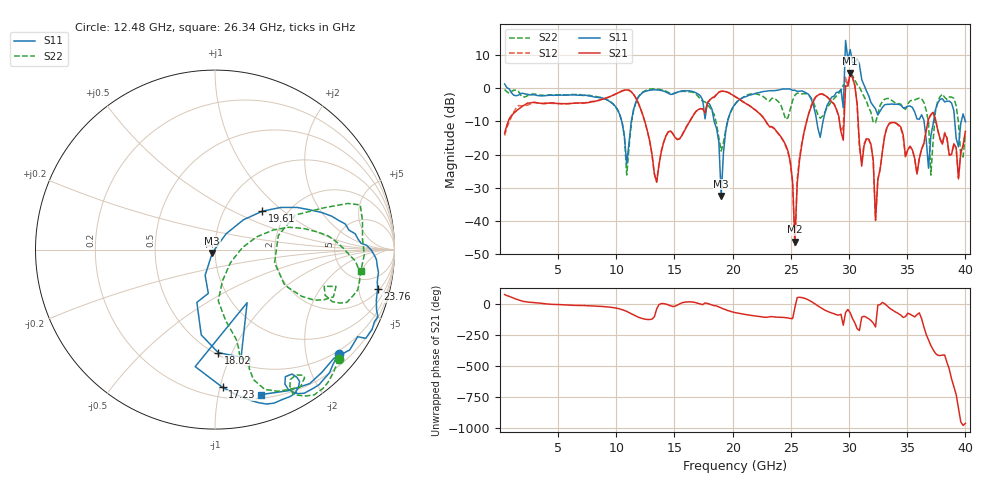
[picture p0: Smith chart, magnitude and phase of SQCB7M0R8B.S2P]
! Network Analyzer HP8722ES.07.66: Jul 25, 2000 Serial No. US39175408
! 26 Oct 2004  10:26:45
! Frequency  S11  S21  S12  S22
# HZ  S  DB R  50
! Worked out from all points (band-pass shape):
!   201 points, 400 MHz to 40 GHz, reference 50 ohm
!   highest |S21| = 4.62 dB at 30.1 GHz (marker M1); lowest = -46.3 dB at 25.35 GHz (marker M2)
!   |S21| within 3 dB of the highest: 29.95 GHz to 30.44 GHz (487.3 MHz wide, 1.61 % of centre)
!   lowest |S11| = -32.5 dB at 19.01 GHz (marker M3), VSWR 1.05, Z = 48.5 - j1.77 ohm
!   |S11| at or under -10 dB: 10.47 GHz to 11.29 GHz (819.6 MHz wide, 7.53 % of centre); 18.41 GHz to 19.57 GHz (1.159 GHz wide, 6.1 % of centre); 36.45 GHz to 37.26 GHz (812.6 MHz wide, 2.2 % of centre)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
!   |S22| runs from -26.2 to 3.9 dB; largest |S21 - S12| = 0.62
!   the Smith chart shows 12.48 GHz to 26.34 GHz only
!   S11 on the Smith chart (normalised r, x): 12.48 GHz: 0.43, -2.67; 17.23 GHz: 0.27, -1.02; 18.02 GHz: 0.52, -0.89; 19.61 GHz: 1.51, +0.73; 23.76 GHz: 2.25, -7.65; 26.34 GHz: 0.23, -1.34
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4e8  1.30 -15.1  -13.48 75.8  -14.23 80.6  -0.38 -7.8
7.132e9  -2.14 -101.7  -4.42 -12.5  -4.51 -14.0  -2.13 -105.2
1.2478e10  -0.91 -40.2  -10.35 -122.8  -10.43 -123.5  -0.73 -41.4
1.3666e10  -0.52 -58.1  -23.20 -5.2  -22.89 -3.4  -0.33 -57.9
1.723e10  -2.29 -86.9  -6.15 0.0  -6.14 0.4  -3.26 -73.9
1.8022e10  -4.82 -88.2  -3.58 -1.9  -3.53 -1.8  -5.74 -76.6
1.9012e10  -32.52 -129.6  -0.91 -32.2  -0.90 -32.3  -18.95 -40.1
1.9606e10  -9.37 39.0  -1.25 -53.8  -1.21 -53.7  -9.33 18.6
2.02e10  -4.85 22.8  -2.54 -69.8  -2.45 -69.5  -4.78 9.9
2.3764e10  -0.61 -13.7  -12.97 -106.3  -13.06 -106.7  -3.52 -24.8
2.5348e10  -0.58 -36.7  -46.33 -29.0  -47.65 -5.7  -2.11 19.1
2.6338e10  -1.44 -72.4  -10.28 40.0  -10.24 39.8  -1.71 -8.2
2.6932e10  -5.02 -116.8  -3.99 9.4  -3.63 9.3  -4.10 -21.4
2.9506e10  -5.93 21.9  -15.68 -171.9  -11.53 -135.9  1.05 25.3
2.9704e10  14.45 -54.2  0.70 -69.0  3.53 -48.2  0.44 -55.6
2.9902e10  8.62 -61.3  0.69 -44.3  0.54 -45.3  1.69 5.2
3.01e10  11.69 -90.8  4.62 -71.8  4.52 -73.2  3.47 -10.1
3.0496e10  7.66 -107.6  0.90 -151.8  0.89 -152.0  2.52 -67.2
3.0694e10  9.00 38.1  -4.62 160.7  -5.03 161.2  1.16 102.3
3.1486e10  -0.69 145.0  -15.25 -108.0  -15.18 -108.0  -3.75 -129.0
3.3466e10  -4.82 -141.0  -10.64 -32.2  -10.53 -32.8  -3.06 -149.5
4e10  -10.07 104.3  -13.03 117.3  -12.88 118.7  -13.88 78.8
